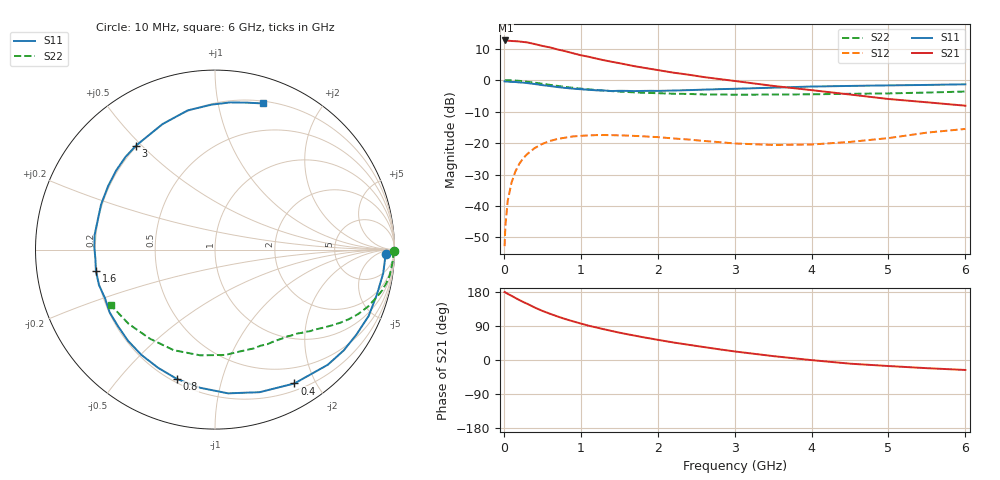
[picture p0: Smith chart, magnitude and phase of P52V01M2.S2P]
! SIEMENS Small Signal Semiconductors
! BFP183
! Si NPN RF Bipolar Junction Transistor in SOT143
! VCE = 2 V  IC = 1.2 mA
! Common Emitter S-Parameters:  March  1996
# GHz  S  MA  R  50
!  f  S11  S21  S12  S22
! GHz  MAG  ANG  MAG  ANG  MAG  ANG  MAG  ANG
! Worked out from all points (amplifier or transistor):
!   36 points, 10 MHz to 6 GHz, reference 50 ohm
!   highest |S21| = 12.6 dB at 20 MHz (marker M1)
!   |S21| within 3 dB of that: start of sweep to 723 MHz
!   unconditionally stable (mu >= 1): 2.394 GHz to end of sweep
!   at 250 MHz: K = 0.11, MSG = 18.5 dB, |S12| = -24.9 dB
!   at 1.4 GHz: K = 0.58, MSG = 11.7 dB, |S12| = -17.5 dB
!   at 6 GHz: K = 1.03, MAG = 2.6 dB, |S12| = -15.5 dB
!   S11 on the Smith chart (normalised r, x): 10 MHz: 33, -17; 400 MHz: 0.29, -1.72; 800 MHz: 0.22, -0.73; 1.6 GHz: 0.20, -0.08; 3 GHz: 0.20, +0.48; 6 GHz: 0.22, +1.36
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0.01  0.9529 -1.4  4.245 179.3  0.0023 84.3  0.9996 -0.6
0.02  0.9487 -3.2  4.264 178.4  0.0048 87.8  0.9909 -1.1
0.05  0.9465 -8.0  4.239 174.6  0.012 89.2  0.9942 -2.8
0.1  0.9363 -15.4  4.177 169.4  0.0236 80.8  0.9883 -5.6
0.15  0.9324 -23.4  4.152 163.8  0.0353 75.7  0.9838 -8.4
0.25  0.9111 -38.0  4.036 153.3  0.057 67.4  0.9598 -13.6
0.3  0.8981 -45.6  3.979 148.7  0.0662 63.2  0.9427 -15.9
0.4  0.8672 -59.3  3.742 138.6  0.0831 55.4  0.9109 -20.3
0.5  0.8325 -72.6  3.493 129.7  0.0969 48.2  0.8752 -24.2
0.6  0.8042 -84.8  3.307 122.0  0.1079 41.9  0.8401 -27.5
0.8  0.7514 -106.3  2.875 108.0  0.1218 31.3  0.7786 -32.7
0.9  0.7312 -115.6  2.668 102.0  0.1275 27.0  0.7549 -34.8
1.1  0.702 -133.7  2.351 90.6  0.1323 19.3  0.7125 -38.7
1.3  0.6833 -149.2  2.07 81.2  0.134 13.0  0.6819 -42.2
1.6  0.674 -169.9  1.758 68.2  0.1315 6.1  0.6483 -46.9
1.9  0.6757 173.0  1.512 56.9  0.126 1.2  0.6247 -51.8
2.2  0.6827 158.4  1.315 46.4  0.1184 -1.9  0.6079 -57.1
3  0.7275 127.2  0.969 22.6  0.0985 -1.4  0.5855 -73.2
3.5  0.758 112.7  0.809 10.3  0.0932 4.8  0.5896 -84.5
4.5  0.808 91.3  0.59 -9.7  0.1042 19.7  0.6058 -112.3
5.5  0.8381 77.6  0.444 -21.6  0.1464 24.6  0.6346 -139.3
6  0.8577 71.7  0.392 -26.3  0.1676 21.6  0.658 -152.0
